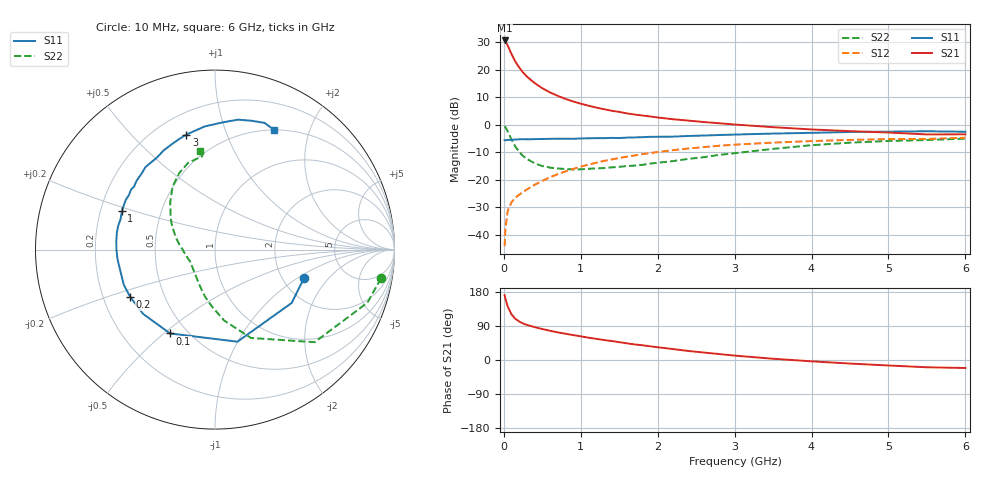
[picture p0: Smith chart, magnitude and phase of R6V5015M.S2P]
! SIEMENS Small Signal Semiconductors
! BFR193
! Si NPN RF Bipolar Junction Transistor in SOT23
! VCE = 0.5 V  IC = 15 mA
! Common Emitter S-Parameters:  May  1996
# GHz  S  MA  R  50
!  f  S11  S21  S12  S22
! GHz  MAG  ANG  MAG  ANG  MAG  ANG  MAG  ANG
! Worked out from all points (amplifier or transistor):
!   36 points, 10 MHz to 6 GHz, reference 50 ohm
!   highest |S21| = 30.6 dB at 10 MHz (marker M1)
!   |S21| within 3 dB of that: start of sweep to 68.98 MHz
!   unconditionally stable (mu >= 1): 521.2 MHz to 2.531 GHz
!   at 250 MHz: K = 0.79, MSG = 21.7 dB, |S12| = -24.5 dB
!   at 1.4 GHz: K = 1.05, MAG = 7.5 dB, |S12| = -12.6 dB
!   at 6 GHz: K = 1.00, MSG = 0.6 dB, |S12| = -4.7 dB
!   S11 on the Smith chart (normalised r, x): 10 MHz: 2.59, -1.14; 100 MHz: 0.40, -0.52; 200 MHz: 0.32, -0.24; 1 GHz: 0.29, +0.18; 3 GHz: 0.32, +0.73; 6 GHz: 0.50, +1.49
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0.01  0.5202 -18.0  33.84 171.1  0.0062 82.6  0.9386 -9.8
0.02  0.5206 -34.8  32.59 162.3  0.0126 75.4  0.8993 -19.2
0.05  0.5281 -76.3  27.49 141.3  0.027 62.7  0.7578 -42.9
0.1  0.53 -118.2  19.12 120.2  0.0391 53.2  0.5312 -67.9
0.15  0.5373 -138.2  13.96 108.7  0.0471 51.5  0.3987 -82.6
0.2  0.5412 -150.7  10.91 101.5  0.0533 52.4  0.3203 -92.7
0.25  0.5447 -159.0  8.846 96.3  0.0598 54.3  0.2694 -101.7
0.3  0.5408 -164.9  7.458 92.6  0.0666 56.1  0.2376 -108.1
0.4  0.5455 -174.2  5.702 86.8  0.0809 58.7  0.1991 -118.8
0.5  0.5494 179.9  4.586 81.7  0.0952 60.4  0.1768 -128.4
0.6  0.552 174.7  3.852 77.2  0.1107 61.1  0.1658 -136.1
0.7  0.5551 169.9  3.34 72.9  0.126 61.4  0.1599 -141.9
0.8  0.5552 166.1  2.941 69.4  0.1414 60.7  0.1565 -147.5
1  0.5611 157.7  2.403 62.4  0.1726 59.6  0.1544 -156.7
1.1  0.5646 154.4  2.208 58.9  0.1881 58.8  0.1579 -160.5
1.6  0.5815 138.6  1.6 44.0  0.262 52.2  0.177 -177.5
2.2  0.6057 122.6  1.254 28.8  0.3437 43.1  0.2178 165.9
3  0.6603 104.0  1.006 11.6  0.4328 29.8  0.3027 144.6
3.5  0.6884 94.8  0.899 3.3  0.4718 21.8  0.3631 133.4
4.5  0.7352 80.0  0.762 -9.4  0.5285 7.9  0.4707 115.1
5.5  0.7581 68.6  0.664 -19.2  0.5491 -4.9  0.5249 97.8
6  0.7434 63.6  0.667 -21.1  0.5789 -8.8  0.558 98.6
